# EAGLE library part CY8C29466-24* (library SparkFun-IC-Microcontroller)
CYPRESS MCU 32K FLASH 2K SRAM 28-SOIC Datasheet SparkFun Products MP3 Trigger (WIG-13720)
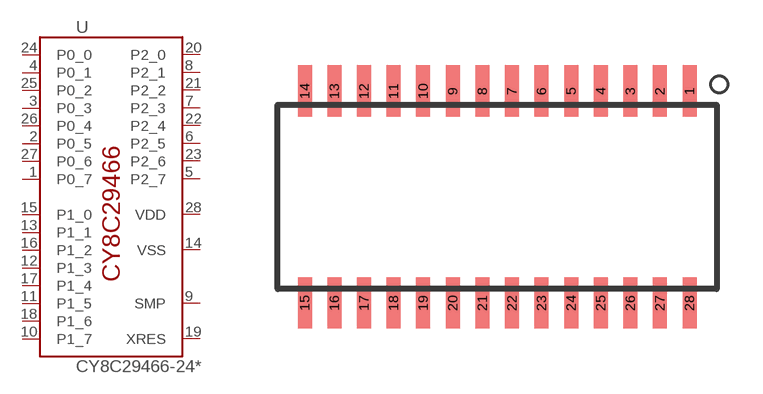
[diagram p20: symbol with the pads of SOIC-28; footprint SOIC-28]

Designator prefix -

## CY8C29466-24 (PROD_ID: IC-08972; VALUE: CY8C29466)  [SOIC-28]
1  P0_7
2  P0_5
3  P0_3
4  P0_1
5  P2_7
6  P2_5
7  P2_3
8  P2_1
9  SMP
10  P1_7
11  P1_5
12  P1_3
13  P1_1
14  VSS  pwr
15  P1_0
16  P1_2
17  P1_4
18  P1_6
19  XRES
20  P2_0
21  P2_2
22  P2_4
23  P2_6
24  P0_0
25  P0_2
26  P0_4
27  P0_6
28  VDD  pwr

## Footprint SOIC-28 (pad centres in mm)
smd 0.6 x 2.2: 1 8.89,4.548; 2 7.62,4.548; 3 6.35,4.548; 4 5.08,4.548; 5 3.81,4.548; 6 2.54,4.548; 7 1.27,4.548; 8 0,4.548; 9 -1.27,4.548; 10 -2.54,4.548; 11 -3.81,4.548; 12 -5.08,4.548; 13 -6.35,4.548; 14 -7.62,4.548; 15 -7.62,-4.548; 16 -6.35,-4.548; 17 -5.08,-4.548; 18 -3.81,-4.548; 19 -2.54,-4.548; 20 -1.27,-4.548; 21 0,-4.548; 22 1.27,-4.548; 23 2.54,-4.548; 24 3.81,-4.548; 25 5.08,-4.548; 26 6.35,-4.548; 27 7.62,-4.548; 28 8.89,-4.548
